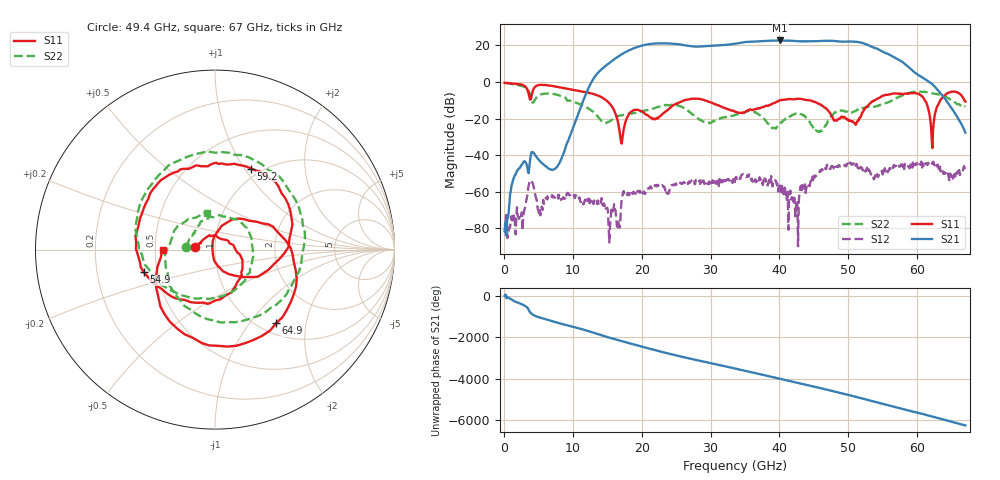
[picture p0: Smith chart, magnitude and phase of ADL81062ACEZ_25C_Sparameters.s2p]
! Analog Devices Inc.
! Device:  ADL81062ACEZ
! Description: GaAs pHEMT Low Noise Amplifier.
! Frequency:  18.00 -  54.00 GHz
! Package:
! Conditions:	Vdd = 3.0 V
!		Idd = 120 mA
!		Temp = +25 C
! Calibration: Board loss de-embedded from S21 magnitude. All other RF measurements reference to RF coaxial connector
! Misc:DB
! Freq(GHz)	S11a(dB)	S11p(deg)	S21a(dB)	S21p(deg)	S12a(dB)	S12p(deg)	S22a(dB)	S22p(deg)
# GHz S  dB  R 50
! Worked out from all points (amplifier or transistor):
!   670 points, 100 MHz to 67 GHz, reference 50 ohm
!   highest |S21| = 22.7 dB at 40.1 GHz (marker M1)
!   |S21| within 3 dB of that: 29.72 GHz to 53.13 GHz (23.41 GHz wide, 56.5 % of centre)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
!   unconditionally stable (mu >= 1): start of sweep to end of sweep
!   at 11.2 GHz: K = 2881.08, MAG = -11.3 dB, |S12| = -65.8 dB
!   at 33.6 GHz: K = 18.10, MAG = 21.1 dB, |S12| = -52.5 dB
!   at 67 GHz: K = 2248.37, MAG = -27.1 dB, |S12| = -46.6 dB
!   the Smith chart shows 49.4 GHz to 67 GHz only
!   S11 on the Smith chart (normalised r, x): 49.4 GHz: 0.80, +0.02; 54.9 GHz: 0.42, -0.13; 59.2 GHz: 0.90, +1.07; 64.9 GHz: 1.19, -1.36; 67 GHz: 0.55, -0.00
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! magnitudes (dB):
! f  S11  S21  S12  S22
! 100 MHz  -0.4  -81.5  -81.1  -0.6
! 1.9 GHz  -1.0  -48.5  -68.5  -1.6
! 3.9 GHz  -9.4  -40.1  -53.6  -8.5
! 5.2 GHz  -1.6  -43.2  -69.5  -7.0
! 7.6 GHz  -2.5  -46.8  -62.6  -6.9
! 11.3 GHz  -5.2  -12.2  -67.6  -12.5
! 15.3 GHz  -11.6  10.5  -87.7  -21.7
! 17.1 GHz  -33.7  15.2  -64.3  -18.2
! 18.7 GHz  -15.6  18.2  -61.2  -17.1
! 22.4 GHz  -19.4  21.1  -56.8  -13.6
! 27.4 GHz  -9.1  19.5  -53.5  -17.7
! 33.6 GHz  -16.4  21.0  -52.5  -17.9
! 40.1 GHz  -9.9  22.7  -56.6  -22.7
! 42.5 GHz  -9.2  22.3  -66.2  -17.3
! 44.7 GHz  -10.3  22.3  -54.7  -23.7
! 49.4 GHz  -19.1  22.1  -45.9  -15.8
! 54.9 GHz  -7.6  16.8  -48.4  -12.2
! 55.9 GHz  -6.9  15.1  -47.8  -11.0
! 59.2 GHz  -6.1  6.7  -44.6  -5.6
! 62.2 GHz  -36.1  -1.2  -44.7  -6.2
! 64.9 GHz  -5.5  -13.7  -51.8  -9.7
! 67 GHz  -10.7  -27.6  -46.6  -13.6
